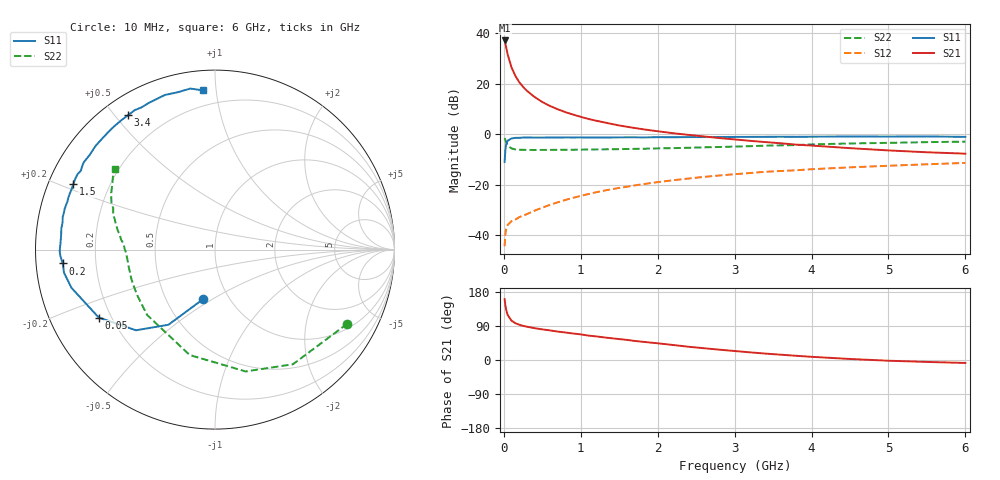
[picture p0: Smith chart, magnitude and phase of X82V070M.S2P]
! SIEMENS Small Signal Semiconductors
! BFP136W
! Si NPN RF Bipolar Junction Transistor in SOT343
! VCE = 2 V  IC = 70 mA
! Common Emitter S-Parameters:  September  1994
# GHz  S  MA  R  50
!  f  S11  S21  S12  S22
! GHz  MAG  ANG  MAG  ANG  MAG  ANG  MAG  ANG
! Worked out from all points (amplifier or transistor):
!   40 points, 10 MHz to 6 GHz, reference 50 ohm
!   highest |S21| = 37.2 dB at 10 MHz (marker M1)
!   |S21| within 3 dB of that: start of sweep to 32.17 MHz
!   unconditionally stable (mu >= 1): 513.6 MHz to 2.917 GHz
!   at 200 MHz: K = 0.64, MSG = 26.7 dB, |S12| = -32.8 dB
!   at 1.5 GHz: K = 1.11, MAG = 10.3 dB, |S12| = -21.2 dB
!   at 6 GHz: K = 0.98, MSG = 1.8 dB, |S12| = -11.3 dB
!   S11 on the Smith chart (normalised r, x): 10 MHz: 0.76, -0.46; 50 MHz: 0.15, -0.26; 200 MHz: 0.08, -0.05; 1.5 GHz: 0.07, +0.22; 3.4 GHz: 0.07, +0.54; 6 GHz: 0.11, +0.92
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0.01  0.2841 -103.5  72.17 160.7  0.0061 70.1  0.8449 -29.3
0.02  0.4927 -121.8  62.3 144.5  0.0105 58.2  0.7723 -55.8
0.03  0.6291 -134.4  52.97 132.9  0.0134 49.2  0.7 -75.9
0.05  0.7503 -149.7  37.98 118.6  0.0161 37.6  0.604 -103.5
0.1  0.8277 -165.1  21.08 103.7  0.0191 33.0  0.5251 -136.1
0.15  0.851 -171.3  14.36 97.1  0.0205 35.5  0.5024 -149.8
0.2  0.8517 -174.8  10.77 93.1  0.0229 38.5  0.4956 -157.3
0.25  0.8623 -177.7  8.694 90.1  0.0245 41.7  0.493 -161.9
0.3  0.8654 -179.5  7.27 87.9  0.0263 44.3  0.4907 -165.1
0.4  0.8611 177.0  5.472 84.0  0.0308 49.5  0.4902 -169.3
0.5  0.8614 174.2  4.363 80.8  0.0353 53.0  0.4906 -172.2
0.6  0.8642 172.2  3.639 78.1  0.0401 55.4  0.4915 -174.0
0.7  0.8626 169.8  3.137 75.0  0.0451 57.6  0.4931 -175.3
0.9  0.8667 166.2  2.457 69.9  0.0553 59.4  0.4955 -177.7
1.1  0.8648 161.8  2.012 64.4  0.0657 60.3  0.5 -179.4
1.5  0.8697 155.2  1.497 55.2  0.0869 60.0  0.5085 177.6
2.2  0.8751 142.9  1.052 39.6  0.1232 55.3  0.5324 172.3
3.2  0.8897 125.9  0.743 20.2  0.1712 46.0  0.5821 163.4
3.4  0.8917 123.0  0.702 16.9  0.1811 43.9  0.5965 161.5
4.5  0.9057 108.0  0.532 2.7  0.2218 33.7  0.6585 151.4
5.5  0.9076 98.7  0.441 -5.1  0.2552 25.6  0.7 144.3
6  0.8899 94.4  0.414 -7.8  0.2714 21.2  0.7151 141.2
